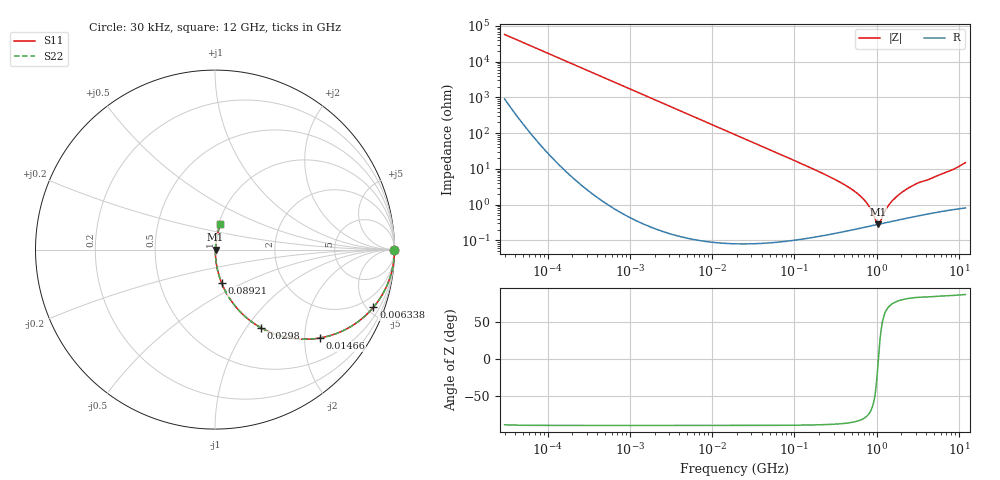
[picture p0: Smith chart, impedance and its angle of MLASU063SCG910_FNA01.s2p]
! MLASU063SCG910_FNA01  S-PARAMETER MODEL  ( General Type )
! Model Generated by TAIYO YUDEN Corporation (http://www.ty-top.com)
! Version 1.0
! TAIYO YUDEN Control No. 130520
! Copyright(c) 2013 TAIYO YUDEN CO.,LTD. All Rights Reserved.
! Product Description (link to TY-COMPAS)
! https://ds.yuden.co.jp/TYCOMPAS/or/detail?pn=MLASU063SCG910JFNA01&u=M
! Products Name : Multilayer Ceramic Capacitors
! Characteristics :
!  Capacitance : 91 pF , Rated Voltage : 50V , TCC : CG / C0G
!  Case Size : 0.6 x 0.3 / 0.024 x 0.012 [mm/inch] , Thickness : 0.3 / 0.012 [mm/inch]
!  (Conditions: Temperature = 25 degC , DC Bias Current/Voltage = 0A / 0V)
! External Node Assignments :
!  1  o---| |---o  2
! GND o---------o GND
! Frequency Range : 0.03MHz  -  12000MHz  [ 401 STEP ]
# MHz S RI R 50
! Freq[MHz].  S11 Real  S11 Imag  S21 Real  S21 Imag  S12 Real  S12 Imag  S22 Real  S22 Imag
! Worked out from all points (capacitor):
!   401 points, 30 kHz to 12 GHz, reference 50 ohm
!   read as one part in series: C = 91.5 pF near 32 kHz
!   lowest |Z| = 285 mohm at 1.035 GHz (marker M1)
!   series resonance near 1.05 GHz, so ESL is about 250 pH
!   S11 on the Smith chart (normalised r, x): 30 kHz: open; 6.338 MHz: 1.00, -5.49; 14.66 MHz: 1.00, -2.37; 29.8 MHz: 1.00, -1.17; 89.21 MHz: 1.00, -0.39; 12 GHz: 1.02, +0.30
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0.03  1 -0.00173  3e-05 0.00173  3e-05 0.00173  1 -0.00173
0.260295  0.9998 -0.015  0.000232 0.015  0.000232 0.015  0.9998 -0.015
2.258455  0.9834 -0.1277  0.0166 0.1277  0.0166 0.1277  0.9834 -0.1277
6.338349  0.8826 -0.3217  0.1174 0.3217  0.1174 0.3217  0.8826 -0.3217
9.639247  0.7647 -0.4239  0.2353 0.4239  0.2353 0.4239  0.7647 -0.4239
14.65919  0.5843 -0.4925  0.4157 0.4925  0.4157 0.4925  0.5843 -0.4925
18.97367  0.4563 -0.4976  0.5437 0.4976  0.5437 0.4976  0.4563 -0.4976
29.80049  0.2539 -0.4346  0.7461 0.4346  0.7461 0.4346  0.2539 -0.4346
48.33933  0.1147 -0.3175  0.8853 0.3175  0.8853 0.3175  0.1147 -0.3175
89.2069  0.037 -0.1861  0.963 0.1861  0.963 0.1861  0.037 -0.1861
164.6252  0.0117 -0.1017  0.9883 0.1017  0.9883 0.1017  0.0117 -0.1017
356.9603  0.00351 -0.0428  0.9965 0.0428  0.9965 0.0428  0.00351 -0.0428
579.0248  0.00254 -0.0208  0.9975 0.0208  0.9975 0.0208  0.00254 -0.0208
774.0045  0.00253 -0.0102  0.9975 0.0102  0.9975 0.0102  0.00253 -0.0102
970.0175  0.00272 -0.00259  0.9973 0.00259  0.9973 0.00259  0.00272 -0.00259
1034.641  0.0028 -0.00046  0.9972 0.00046  0.9972 0.00046  0.0028 -0.00046
1103.571  0.0029 0.00156  0.9971 -0.00156  0.9971 -0.00156  0.0029 0.00156
1428.372  0.00339 0.0097  0.9966 -0.0097  0.9966 -0.0097  0.00339 0.0097
1848.769  0.00408 0.0183  0.9959 -0.0183  0.9959 -0.0183  0.00408 0.0183
2722.352  0.00563 0.0335  0.9944 -0.0335  0.9944 -0.0335  0.00563 0.0335
7890.678  0.0148 0.0875  0.9852 -0.0875  0.9852 -0.0875  0.0148 0.0875
12000  0.0297 0.1447  0.9703 -0.1447  0.9703 -0.1447  0.0297 0.1447
